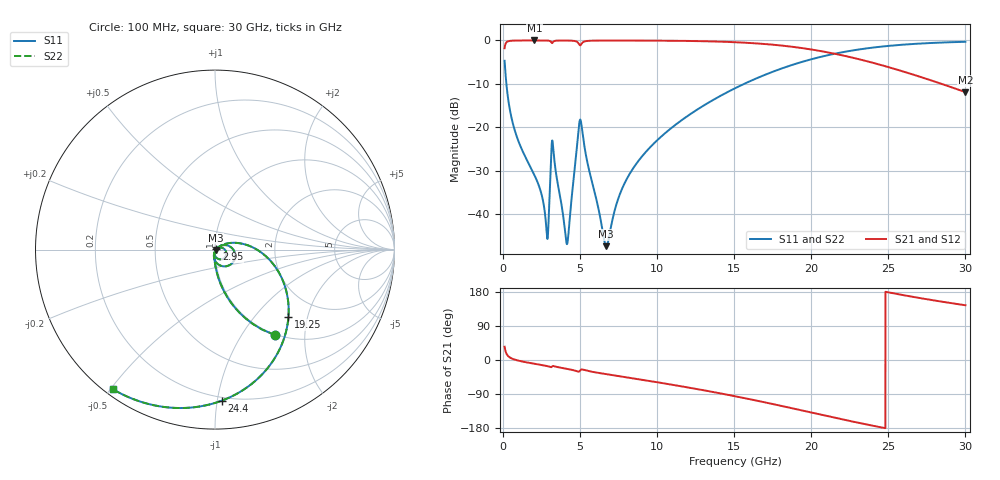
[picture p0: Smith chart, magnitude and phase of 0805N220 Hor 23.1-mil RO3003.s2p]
# GHz S MA R 50
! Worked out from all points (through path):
!   3201 points, 100 MHz to 30 GHz, reference 50 ohm
!   highest |S21| = -0.02 dB at 2.034 GHz (marker M1); lowest = -11.9 dB at 30 GHz (marker M2)
!   group delay of S21, straight-line fit = 21.2 ps
!   lowest |S11| = -47.3 dB at 6.697 GHz (marker M3), VSWR 1.01, Z = 50.4 - j0.249 ohm
!   |S11| at or under -10 dB: 214.8 MHz to 15.64 GHz (15.43 GHz wide, 195 % of centre)
!   |S22| runs from -47.3 to -0.3 dB; largest |S21 - S12| = 0
!   S11 on the Smith chart (normalised r, x): 100 MHz: 0.99, -1.42; 2.95 GHz: 1.02, +0.00; 19.25 GHz: 1.41, -1.53; 24.4 GHz: 0.18, -1.03; 30 GHz: 0.02, -0.51
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0.1  0.5824 -54.9  0.8124 35.1  0.8124 35.1  0.5824 -54.9
0.3335938  0.2094 -79.7  0.9773 10.2  0.9773 10.2  0.2094 -79.7
0.7166875  0.09796 -88.0  0.9944 1.5  0.9944 1.5  0.09796 -88.0
2.034156  0.02827 -97.0  0.9981 -9.9  0.9981 -9.9  0.02827 -97.0
2.501344  0.01684 -96.4  0.9978 -13.2  0.9978 -13.2  0.01684 -96.4
2.800344  0.007222 -76.0  0.9963 -15.5  0.9963 -15.5  0.007222 -76.0
2.949844  0.008146 9.7  0.9926 -16.9  0.9926 -16.9  0.008146 9.7
3.127375  0.05136 4.3  0.9524 -18.9  0.9524 -18.9  0.05136 4.3
3.248844  0.0595 -65.3  0.9602 -15.8  0.9602 -15.8  0.0595 -65.3
4.033719  0.006054 -69.2  0.9957 -22.5  0.9957 -22.5  0.006054 -69.2
4.173875  0.004665 -17.3  0.9952 -23.6  0.9952 -23.6  0.004665 -17.3
4.884  0.08937 9.0  0.9294 -30.7  0.9294 -30.7  0.08937 9.0
5.089563  0.1064 -61.7  0.9125 -24.9  0.9125 -24.9  0.1064 -61.7
6.696688  0.004302 -35.0  0.9955 -37.3  0.9955 -37.3  0.004302 -35.0
7.930063  0.02361 35.3  0.9956 -45.2  0.9956 -45.2  0.02361 35.3
10.06978  0.07294 27.5  0.9928 -59.2  0.9928 -59.2  0.07294 27.5
15.05  0.2814 -6.8  0.953 -95.6  0.953 -95.6  0.2814 -6.8
19.24534  0.5555 -42.6  0.8228 -131.7  0.8228 -131.7  0.5555 -42.6
20.03956  0.6091 -49.7  0.784 -138.9  0.784 -138.9  0.6091 -49.7
24.40309  0.8424 -87.4  0.5283 -176.8  0.5283 -176.8  0.8424 -87.4
25.01978  0.8644 -92.3  0.492 178.4  0.492 178.4  0.8644 -92.3
30  0.9636 -126.1  0.2542 144.5  0.2542 144.5  0.9636 -126.1
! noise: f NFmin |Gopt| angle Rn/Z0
0.1  0.0005931  0.8967  0.8136  0.001254
3.417  0.01338  0.8486  19.34  0.01828
6.743  0.01271  0.7147  37.58  0.007907
10.06  0.01537  0.6681  54.6  0.007097
13.39  0.01986  0.6697  70.44  0.007863
16.7  0.02545  0.6867  85.06  0.008817
20.03  0.03271  0.7142  98.75  0.009937
23.35  0.04257  0.7498  111.7  0.01128
26.67  0.05687  0.7921  124.4  0.01289
30  0.07897  0.8383  136.9  0.01462
